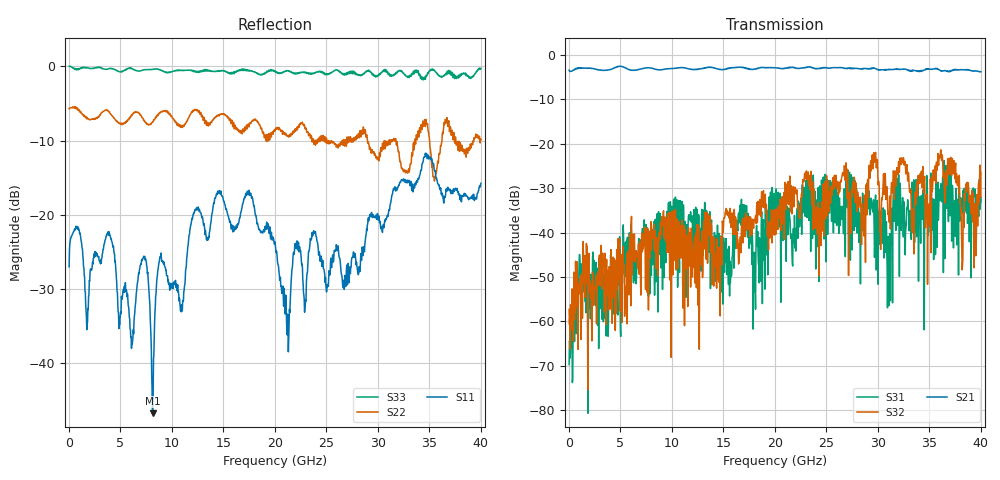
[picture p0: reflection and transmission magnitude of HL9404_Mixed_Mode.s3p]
! HYPERLABS, INC. 03/12/2021
! MIXED MODE  S-PARAMETERS
! CALCULATED FROM A MEASURED DATA S3P FILE
# GHZ S RI R 50.0
! FREQ.GHZ S11 SSD12 SSC12
! SDS21 SDD22 SDC22
! SCS21 SCD22 SCC22
!; PortSelection: Port_123
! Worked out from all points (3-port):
!   1143 points, 35 MHz to 40.01 GHz, reference 50 ohm
!   strongest paths, dB at 35 MHz, 10.01 GHz, 20.02 GHz, 30.03 GHz, 40.01 GHz:
!     S21: -3.5, -3.1, -2.9, -3.3, -3.8
!     S32: -57.3, -37.8, -34.7, -29.3, -26.4
!     S31: -69.7, -34.1, -34.6, -51.6, -33.1
!   lowest |S11| = -46.8 dB at 8.155 GHz (marker M1), VSWR 1.01, Z = 49.8 + j0.397 ohm
!   |S11| at or under -10 dB: start of sweep to end of sweep
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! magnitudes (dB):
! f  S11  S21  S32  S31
! 35 MHz  -27.0  -3.5  -57.3  -69.7
! 1.225 GHz  -23.7  -3.0  -49.4  -56.7
! 8.155 GHz  -46.8  -3.1  -41.3  -47.2
! 16.8 GHz  -19.1  -2.8  -38.0  -35.8
! 18.02 GHz  -19.1  -3.3  -37.4  -44.4
! 20.02 GHz  -23.6  -2.9  -34.7  -34.6
! 21.59 GHz  -28.8  -2.9  -29.5  -40.8
! 22.71 GHz  -28.6  -3.0  -28.1  -32.2
! 31.05 GHz  -19.6  -3.3  -35.9  -42.3
! 40.01 GHz  -15.8  -3.8  -26.4  -33.1
